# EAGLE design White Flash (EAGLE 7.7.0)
DESIGNER: A. Stummer; GROUP: R. Marjoribanks Labs; RELEASE_DATE: 2017 July; REV: A; TITLE: White Flash
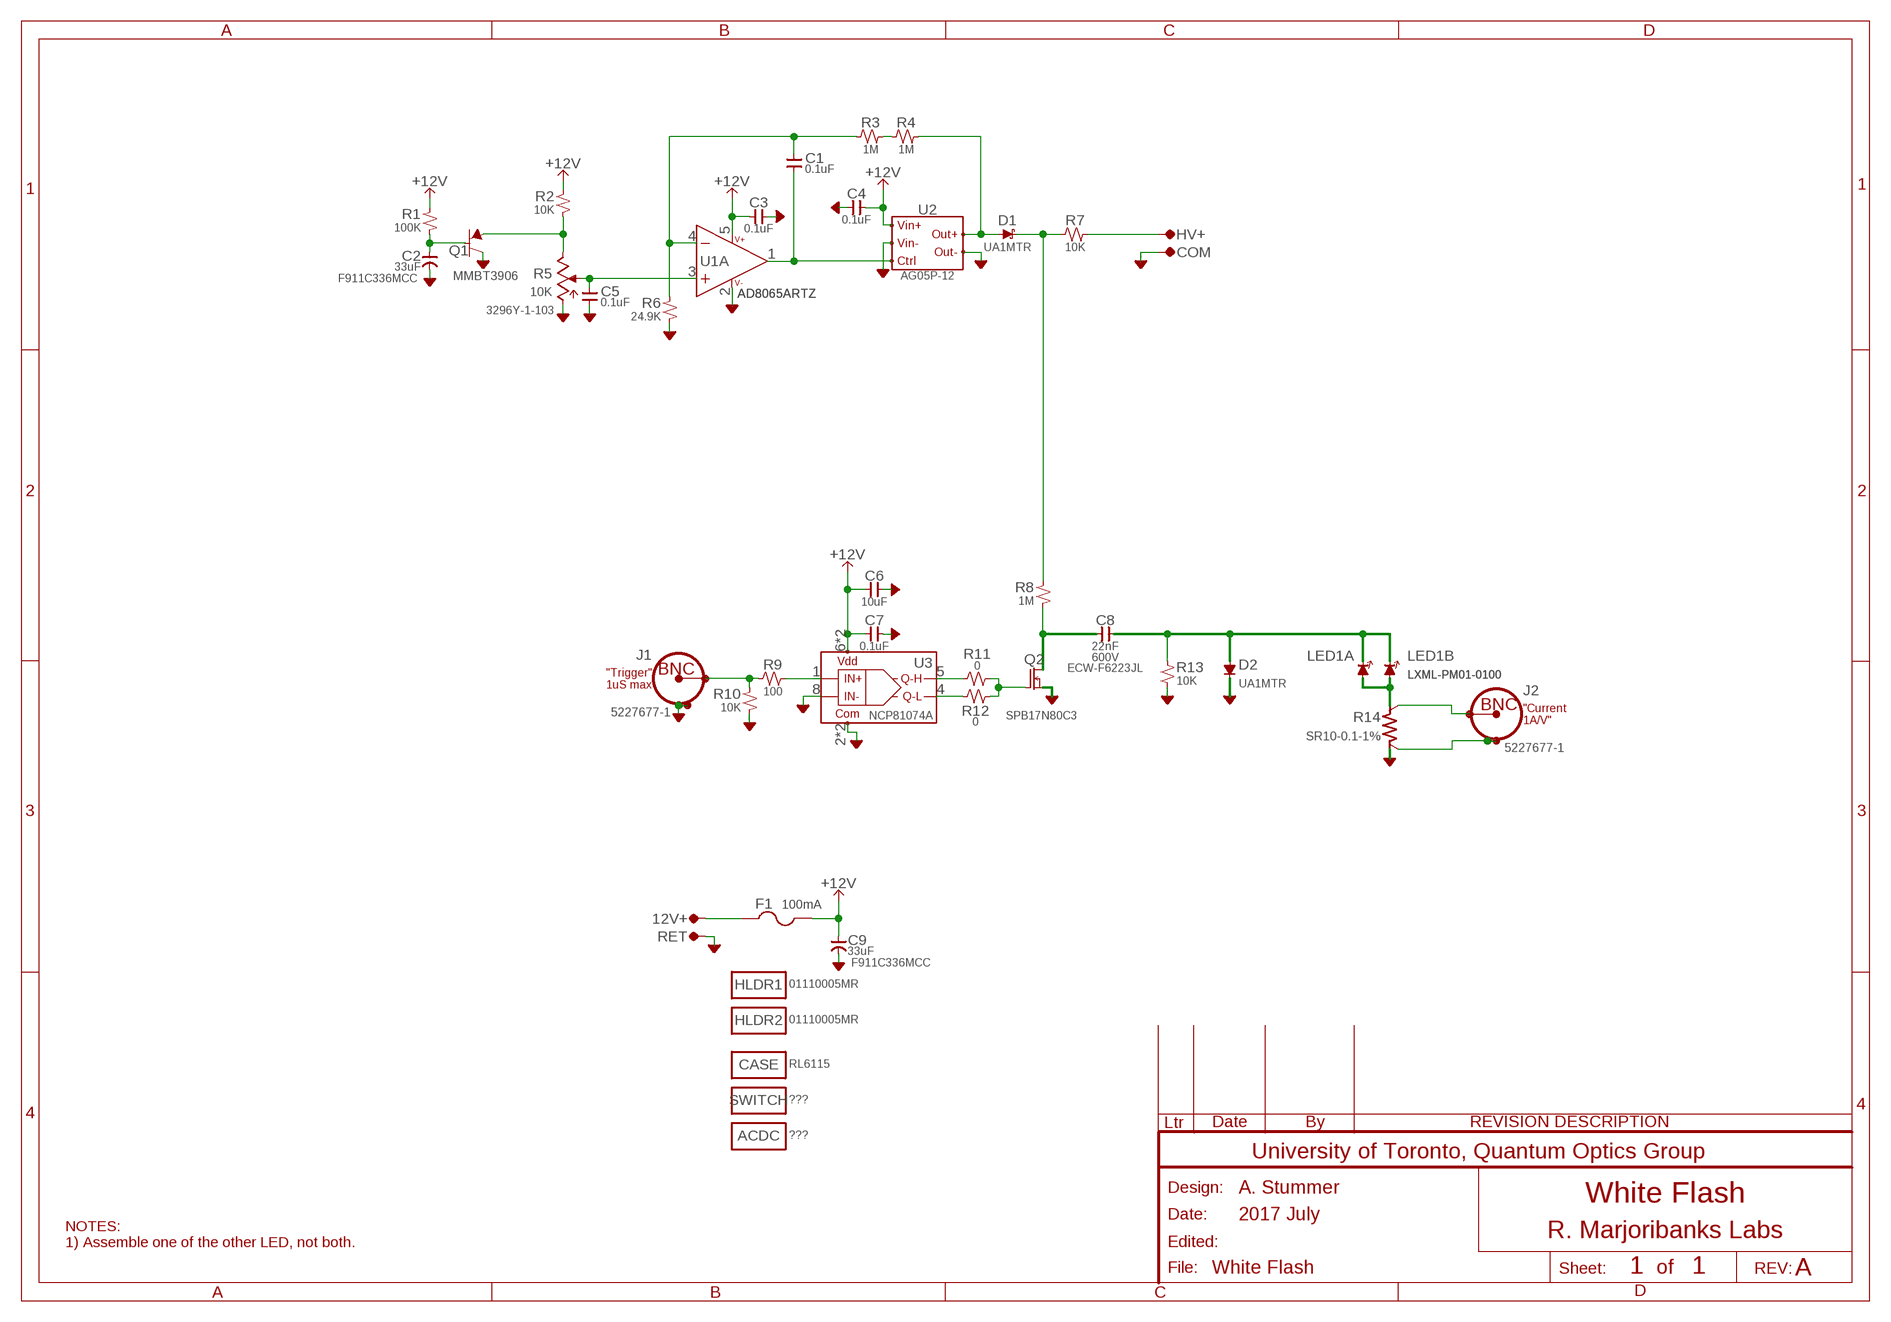
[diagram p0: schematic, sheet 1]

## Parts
12V+  TP-0.042B  [TP-0.042B]
ACDC  ???  MISC  [MISC]
C1  0.1uF  CAP-V-0805  [2012(0805)]
C2  33uF  CAP-POL--NICHICON_F91_C  [CAP:NICHICON_F91_C]
C3  0.1uF  CAP-H-0805  [2012(0805)]
C4  0.1uF  CAP-H-0805  [2012(0805)]
C5  0.1uF  CAP-V-0805  [2012(0805)]
C6  10uF  CAP-H-0805  [2012(0805)]
C7  0.1uF  CAP-H-0805  [2012(0805)]
C8  22nF  CAP-H--PASSIVE,10MM  [PASSIVE_10MM]
C9  33uF  CAP-POL--NICHICON_F91_C  [CAP:NICHICON_F91_C]
CASE  RL6115  MISC  [MISC]
COM  TP-0.042B  [TP-0.042B]
D1  UA1MTR  DIODE,SCHOTTKY-SMA  [EIA-A(SMA)]
D2  UA1MTR  DIODE,GENERIC-SMA  [EIA-A(SMA)]
F1  100mA  FUSE-5X20-4  [FUSE]
HLDR1  01110005MR  MISC  [MISC]
HLDR2  01110005MR  MISC  [MISC]
HV+  TP-0.042B  [TP-0.042B]
J1  5227677-1  CONN:BNCTYPE3HORIZ  [CONN:BNC-AMP-TYPE3HORIZ]
J2  5227677-1  CONN:BNCTYPE3HORIZ  [CONN:BNC-AMP-TYPE3HORIZ]
LED1A  LXML-PM01-0100  LED-LUMILED_REBEL  [LED_LUMILED_REBEL]
LED1B  LXML-PM01-0100  LED-LUMILED_REBEL  [LED_LUMILED_REBEL]
Q1  MMBT3906  BJT-PNP-SOT23  [SOT23]
Q2  SPB17N80C3  MOSFET-N-TO263  [TO263]
R1  100K  R-V-0805  [2012(0805)]
R2  10K  R-V-0805  [2012(0805)]
R3  1M  R-H-0805  [2012(0805)]
R4  1M  R-H-0805  [2012(0805)]
R5  10K  POT-BOURNS_3296Y  [BOURNS:3296Y]
R6  24.9K  R-V-0805  [2012(0805)]
R7  10K  R-H-0805  [2012(0805)]
R8  1M  R-V-0805  [2012(0805)]
R9  100  R-H-0805  [2012(0805)]
R10  10K  R-V-0805  [2012(0805)]
R11  0  R-H-0805  [2012(0805)]
R12  0  R-H-0805  [2012(0805)]
R13  10K  R-V-0805  [2012(0805)]
R14  SR10-0.1-1%  R-SENSE-CADDOCK_SR10  [RESISITOR,CURRENTSENSE,CADDOCK_SR10]
RET  TP-0.042B  [TP-0.042B]
SWITCH  ???  MISC  [MISC]
U1  AD8065ARTZ  OPAMP-SOT23-5  [SOT23-5]
U2  AG05P-12  DC-DC,AG-SERIES-AG(TO2KV)  [DC-DC,AG-SERIES(TO2KV)]
U3  NCP81074A  LOGIC,FET_DRIVER(NCP81074)-SOIC8  [SOIC-8]

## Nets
+12V: C3.2 C4.2 C6.1 C7.1 C9.+(POS) F1.2A F1.2B(2A) R1.2 R2.2 U1.5(B:V++) U2.IN+ U3.6(VDD) U3.7(VDD)
AGND: C2.-(NEG) C3.1 C4.1 C5.1 C6.2 C7.2 C9.-(NEG) COM.TP D2.K(C) J1.SHIELD1 J1.SHIELD2 Q1.2(E) Q2.3(S) R5.CCW R6.1 R10.1 R13.1 R14.CUR2(CURRENT2) RET.TP U1.2(B:V-) U2.HV-(OUT-) U2.IN- U3.2(COM) U3.3(COM) U3.8(IN-)
N$1: R11.1 U3.5(Q-H)
N$2: R9.2 U3.1(IN+)
N$3: J1.CONDUCTOR R9.1 R10.2
N$4: R12.1 U3.4(Q-L)
N$5: Q2.1(G) R11.2 R12.2
N$6 [HV]: D1.K(C) R7.1 R8.2
N$7 [power]: C8.1 Q2.2(D) Q2.4(D) R8.1
N$8: C1.2 R3.1 R6.2 U1.4(A:-IN)
N$9 [HV]: D1.A R4.2 U2.HV+(OUT+)
N$10: C1.1 U1.1(A:OUT) U2.CTRL
N$12: C5.2 R5.W U1.3(A:+IN)
N$13: Q1.3(C) R2.1 R5.CW
N$14: C2.+(POS) Q1.1(B) R1.1
N$15 [power]: C8.2 D2.A LED1A.K(C) LED1B.K(C) R13.2
N$16 [HV]: HV+.TP R7.2
N$17 [Pwr-LV]: LED1A.A LED1B.A R14.CUR1(CURRENT1)
N$18 [HV]: R3.2 R4.1
N$19 [Pwr-LV]: J2.CONDUCTOR R14.SEN1(SENSE1)
N$20: J2.SHIELD1 J2.SHIELD2 R14.SEN2(SENSE2)
N$22: 12V+.TP F1.1A F1.1B(1A)

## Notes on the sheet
- "Trigger"
  1uS max
- "Current
  1A/V"
- NOTES:
  1) Assemble one of the other LED, not both.

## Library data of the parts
12V+ COM HV+ RET = QuantumOptics:TP: Testpoint, single pin or single socket, either SMT pad, small hole or loop style TP such as Keystone 5002K (0.042").
ACDC CASE HLDR1 HLDR2 SWITCH = QuantumOptics:MISC: Miscellaneous Part, just a placeholder for miscellaeous parts
C1 C5 = QuantumOptics:CAP-V-: Cap, SMT and Through-hole, 0402 and up.
C2 C9 = QuantumOptics:CAP-POL-: Capacitor, Polarized, SMT 0805 and up, probably tantalum.; PN: F911C336MCC
C3 C4 C6 C7 = QuantumOptics:CAP-H-: Cap, SMT and Through-hole, 0402 and up.
C8 = QuantumOptics:CAP-H-: Cap, SMT and Through-hole, 0402 and up.; PN: ECW-F6223JL; V: 600V
D1 = QuantumOptics:DIODE,SCHOTTKY: Schottky Diode, general purpose.
D2 = QuantumOptics:DIODE,GENERIC: Diode, Generic, plain old vanilla diodes.
F1 = QuantumOptics:FUSE: Fuse
J1 J2 = QuantumOptics:CONN:BNC: BNC PCB, horizontal or vertical, e.g. Horiz: Amp (5)227677-1, nut 1-329631-2, shoulder washer 330620, vert isolated 5227222-6, http://catalog.tycoelectronics.com/TE/bin/TE.Connect?C=1&M=BYPN&TCPN=5227222-6&RQPN=5227222-6 ...
LED1A LED1B = QuantumOptics:LED: LED or laser
Q1 = QuantumOptics:BJT-PNP: PNP BJT, generic, p/n defined by VALUE field. E.g. Fairchild MMBT3906 (abs max 40V, 200mA. hFE>80@10mA.
Q2 = QuantumOptics:MOSFET-N: Mosfet, N-Channel, generic enhancement mode N-FET, such as 2N7002 in SOT-23.
R1 R2 R6 R8 R10 R13 = QuantumOptics:R-V-*: Resistor, SMT & Through-Hole, vertical symbol
R3 R4 R7 R9 R11 R12 = QuantumOptics:R-H-*: Resistor, SMT & Through-Hole, horizontal symbol
R5 = QuantumOptics:POT: Pot, regular or trimpot; PN: 3296Y-1-103
R14 = QuantumOptics:R-SENSE: Current sense resistor, 4-terminal. e.g. Ohmite series 60, http://www.ohmite.com/cgi-bin/showpage.cgi?product=60-4_series
U1 = QuantumOptics:OPAMP: Op Amp, generic, pick the right package. e.g. AD8605: SOT-23-5, RRIO, 10MHz, Ib = 1pA, Vio < 65uV, 2.7-5.5V.
U2 = QuantumOptics:DC-DC,AG-SERIES: DC-DC converter, HV #1, based on XP-Emco AG series, 100V-6KV, 1-1.5W
U3 = QuantumOptics:LOGIC,FET_DRIVER(NCP81074): FET Driver, based on NCP81074A/B, 10A 4nS

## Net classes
0 default: width 0.203 mm, drill 0.508 mm, clearance 0.203 mm
1 power: width 2.54 mm, drill 0.508 mm, clearance 2.032 mm
2 HV: width 0.203 mm, drill 0.508 mm, clearance 2.032 mm
3 Pwr-LV: width 2.54 mm, drill 0.508 mm, clearance 0.508 mm

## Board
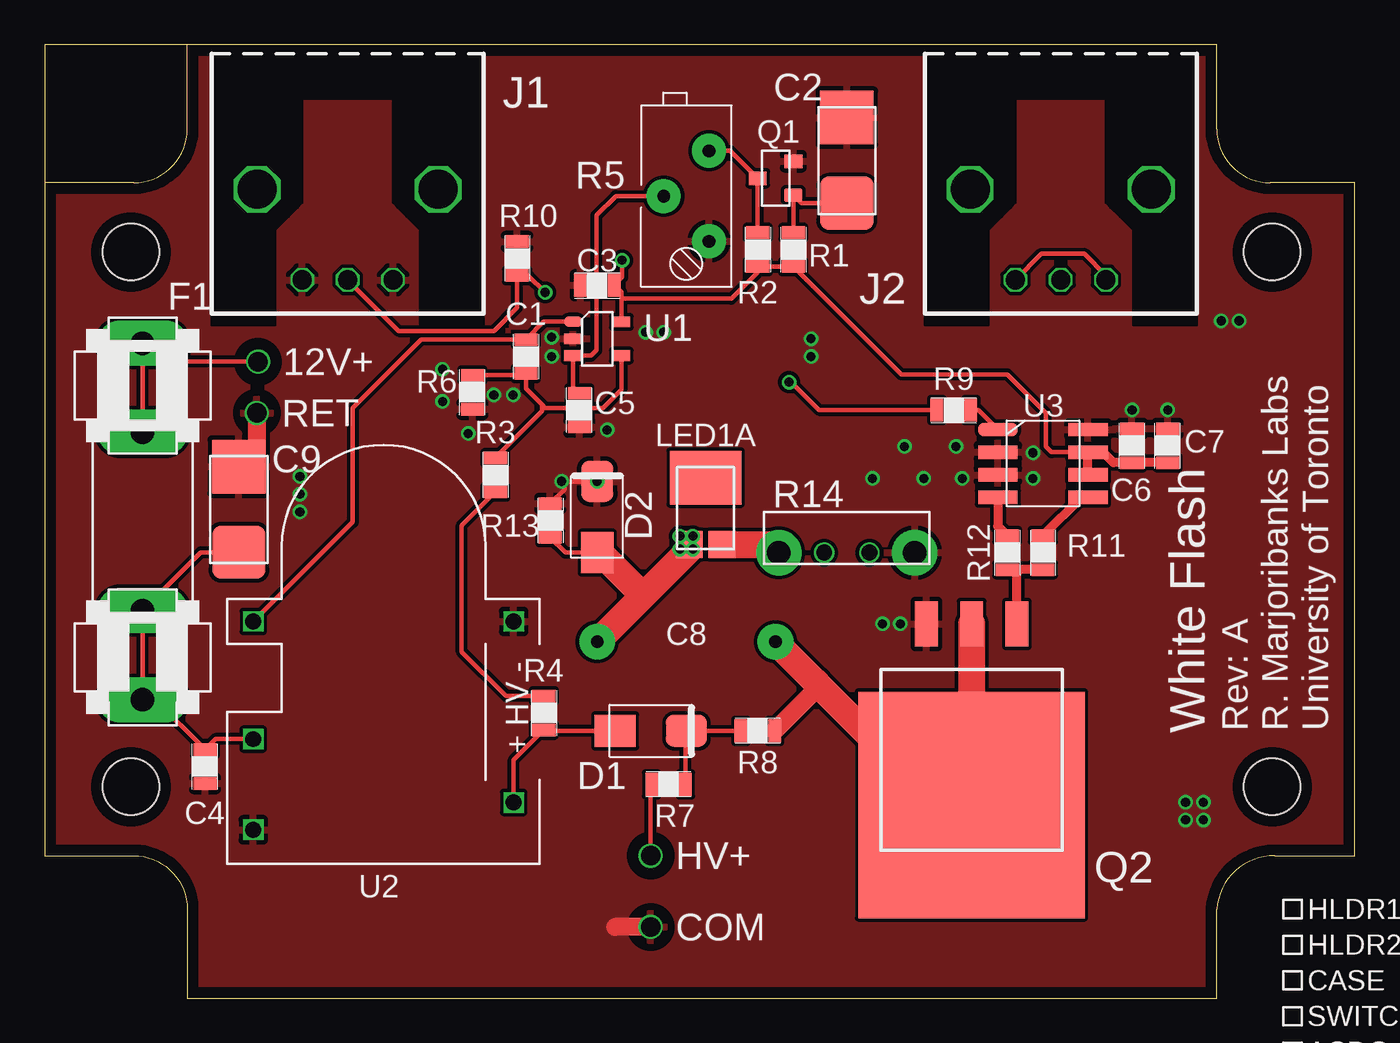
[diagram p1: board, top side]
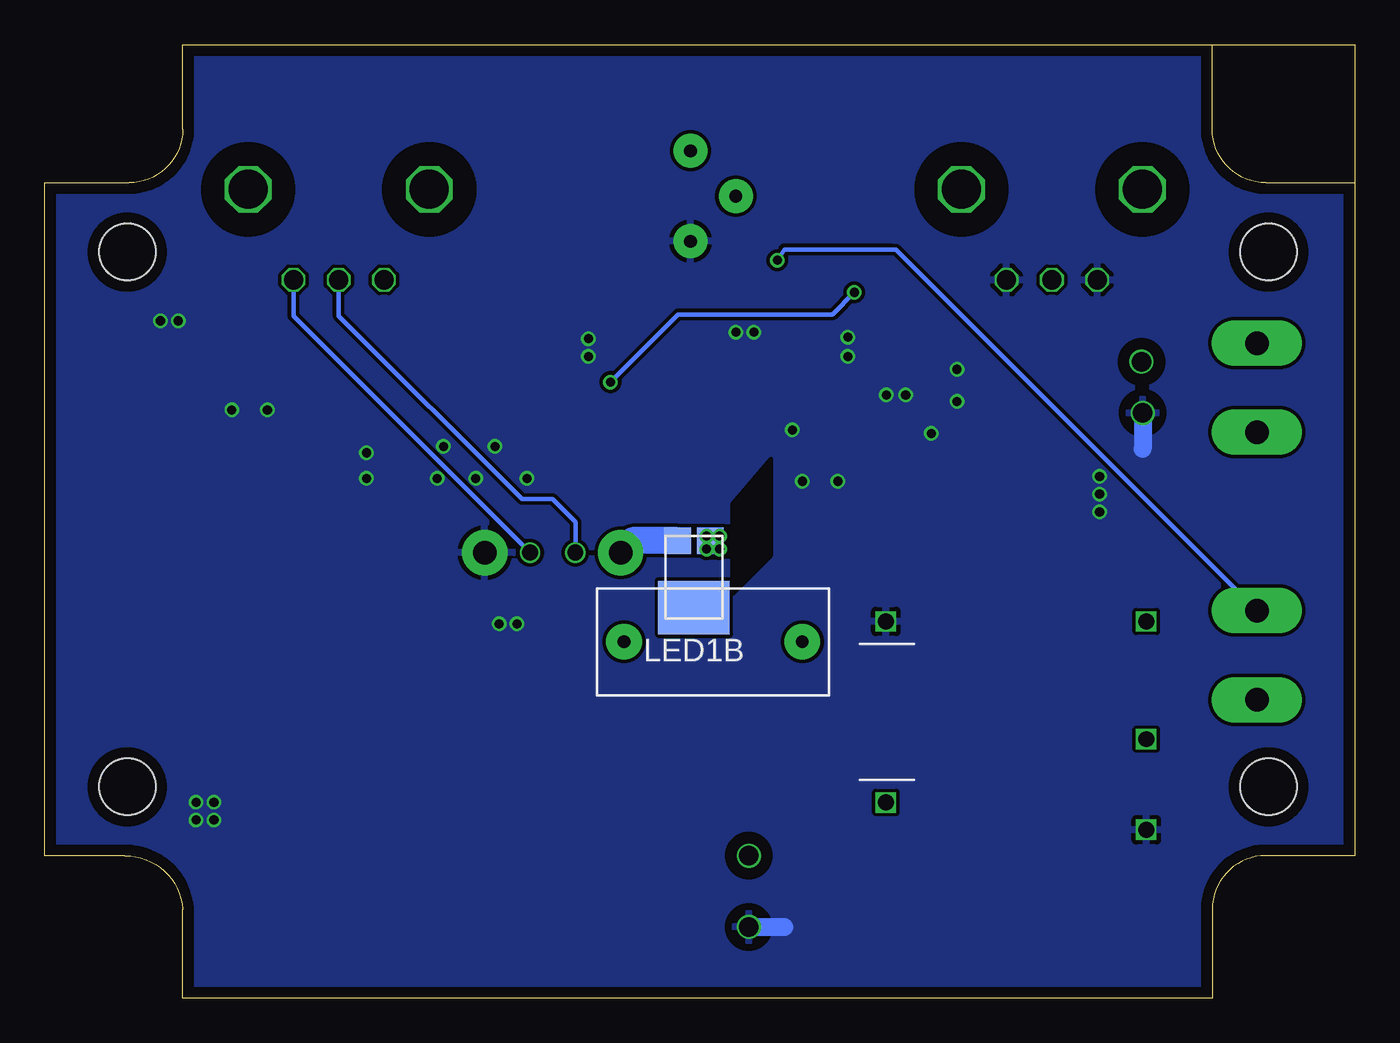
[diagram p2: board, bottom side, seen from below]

Size 73.5 x 53.5 mm. Coordinates in mm from the lower left corner, seen from the top.
Outline: 0,45.75 0,53.5 65.75,53.5 65.75,48.75 arc90 68.75,45.75 73.5,45.75 73.5,8 69,8 arc86 65.75,5 65.75,0 8,0 8,5 arc90 5,8 0,8 0,45.75
Outline: 8,53.5 8,48.75 arc-90 5,45.75 0,45.75
Copper layers (1+16): Top 0.035mm / dielectric 1.5mm / Bottom 0.035mm
Design rules "~DRC for APC, 2-layer": minimum track width 0.18mm, minimum drill 16mil, track to track 0.18mm, track to pad 0.18mm, pad to pad 0.18mm, via to via 0.18mm, smd to smd 0mil, copper to edge 25mil, drill to drill 5mil, minimum pad ring 5mil, minimum via ring 6mil, stop-mask expansion 4mil, vias tented up to drill 0mil, thermal gap 10mil
Holes 3.17 mm at 4.85,11.86 4.85,41.86 68.86,41.86 68.86,11.86
bRestrict: area 32.8,22.7 to 34.9,30.2

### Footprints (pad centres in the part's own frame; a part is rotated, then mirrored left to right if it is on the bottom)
TP-0.042B = drill 1.092: TP 0,0
2012(0805) = smd 0.7 x 1.3: 1 -0.95,0; 2 0.95,0
CAP:NICHICON_F91_C = smd 3 x 3: + -2.4,0; - 2.4,0
PASSIVE_10MM = drill 0.711 pad 2: 1 -5,0; 2 5,0
EIA-A(SMA) = smd 2.3 x 1.8: A -2,0; K 2,0
FUSE = drill 1.321 pad 2.54 long: 1A -10,0; 1B -5,0; 2A 10,0; 2B 5,0
CONN:BNC-AMP-TYPE3HORIZ = drill 1.067 octagon: CONDUCTOR 0,-12.7; SHIELD1 -2.54,-12.7; SHIELD2 2.54,-12.7 | drill 2.184 octagon: P$1 -5.08,-7.62; P$2 5.08,-7.62
LED_LUMILED_REBEL = smd 1.5 x 1.5: A 0.92,0.25; K -0.92,0.25 | smd 4 x 3: THERM 0,4
SOT23 = smd 0.75 x 1: 1 -0.95,-1; 2 0.95,-1; 3 0,1
TO263 = smd 1.27 x 2.54: 1 -2.54,0; 2 0,0; 3 2.54,0 | smd 12.7 x 12.7: 4 0,10.16
BOURNS:3296Y = drill 0.711 pad 1.905: CCW 2.54,1.27; CW -2.54,1.27; W 0,-1.27
RESISITOR,CURRENTSENSE,CADDOCK_SR10 = drill 1.321 pad 2.54: CUR1 -3.81,0; CUR2 3.81,0 | drill 0.889: SEN1 -1.27,0; SEN2 1.27,0
SOT23-5 = smd 0.6 x 1: 1 -0.95,-1.35; 2 0,-1.35; 3 0.95,-1.35; 4 0.95,1.35; 5 -0.95,1.35
DC-DC,AG-SERIES(TO2KV) = drill 0.889 square: CTRL 0,7.303; HV+ -10.16,-7.303; HV- 0,-7.303; IN+ -6.604,7.303; IN- -11.684,7.303
SOIC-8 = smd 0.75 x 2.2: 1 -1.905,-2.532; 2 -0.635,-2.532; 3 0.635,-2.532; 4 1.905,-2.532; 5 1.905,2.532; 6 0.635,2.532; 7 -0.635,2.532; 8 -1.905,2.532

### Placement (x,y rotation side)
12V+  11.97,35.71 0 top
ACDC  70,-3 0 top
C1  27,36 270 top
C2  45,47 90 top
C3  31,40 0 top
C4  9,13 90 top
C5  30,33 90 top
C6  61,31 90 top
C7  63,31 90 top
C8  36,20 0 bottom
C9  10.9,27.42 90 top
CASE  70,1 0 top
COM  34,4 0 top
D1  34,15 0 top
D2  31,27 90 top
F1  5.5,26.75 270 top
HLDR1  70,5 0 top
HLDR2  70,3 0 top
HV+  34,8 0 top
J1  17,53 0 top
J2  57,53 0 top
LED1A  37.08,25.2 0 top
LED1B  37.08,25.92 180 bottom
Q1  41,46 90 top
Q2  52,21 180 top
R1  42,42 270 top
R2  40,42 270 top
R3  25.28,29.36 270 top
R4  28,16 270 top
R5  36,45 270 top
R6  24,34 90 top
R7  35,12 180 top
R8  40,15 180 top
R9  51,33 0 top
R10  26.5,41.5 270 top
R11  56,25 270 top
R12  54,25 270 top
R13  28.36,26.8 270 top
R14  45,25 0 top
RET  11.91,32.83 0 top
SWITCH  70,-1 0 top
U1  31,37 270 top
U2  19.01,21.14 90 top
U3  56,30 270 top
U$24  [CASE,HAMMOND_RL6105_RL6115]  0,0 90 bottom

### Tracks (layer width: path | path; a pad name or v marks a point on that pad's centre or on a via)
+12V  (via drill 0.51)
  Top 0.254: U1.5 32.35,39.24 | 32.35,39.24 32.35,39.6 C3.2 32.4,40.45 v32.4,41.4 | 32.35,39.24 38.52,39.24 40,40.72 R2.2 R1.2 48.05,35 54,35 56.16,32.84 56.16,30.96 56.48,30.64 U3.7 | U2.IN+ 9.59,14.54 C4.2 6.2,16.75 F1.2A F1.2B 8.77,25.02 C9.+
  Top 0.5: U3.6 U3.7 58.57,30.6 59.4,30.6 59.95,30.05 C6.1 C7.1
  Bottom 0.25: 20.15,36.4 25.75,42 26,42
  Bottom 0.254: F1.2B 20.15,36.4 | 26,42 32,42 v32.4,41.4
AGND  (via drill 0.51)
  Top 0.254: 11.91,30.83 C9.- | R13.1 29.16,28.55 29.16,28.8 29.36,29 D2.K
  Top 1: COM.TP 32,4 | RET.TP 11.91,30.83
  Bottom 1: RET.TP 11.91,30.83 | COM.TP 32,4
  other vias: 43,36 43,37 48,21 47,21 61,33 63,33 55.44,30.6 55.44,29.16 51.48,29.16 51.12,30.96 49.32,29.16 46.44,29.16 48.24,30.96 65,10 65,11 64,11 64,10 66,38 67,38 31,29 31.56,31.88 29,29 33.72,37.36 34.72,37.36 28.44,37.08 28.44,36 22.32,35.28 22.32,33.48 25.2,33.84 26.28,33.84 23.76,31.68 14.32,29.28 14.32,28.28 14.32,27.28
  pour Bottom: 0,0 73.5,0 73.5,53.5 0,53.5
  pour Top: 0,0 73.5,0 73.5,53.5 0,53.5
N$1
  Top 0.5: U3.5 58.15,28.09 R11.1
N$2
  Top 0.254: R9.2 52.37,33 U3.1
N$3  (via drill 0.51)
  Top 0.254: 26.37,40.68 R10.2 | R10.2 27.13,40.55 v28.08,39.6 | R9.1 43.44,33 41.88,34.56 v41.76,34.56 | J1.CONDUCTOR 19.86,37.44 25.2,37.44 26.5,38.74 R10.2
  Bottom 0.254: v28.08,39.6 29.32,38.36 37.96,38.36 v41.76,34.56
N$4
  Top 0.5: U3.4 53.47,26.48 R12.1
N$5
  Top 0.5: R11.2 54.72,24.05 | 54.72,24.05 R12.2 | Q2.1 54.54,23.87 54.72,24.05
N$6
  Top 0.254: R7.1 35.95,14.95 D1.K R8.2
N$7
  Top 1: 50.16,10.84 Q2.4 | R8.1 43.28,17.33 43.28,17.72
  Top 1.5: C8.1 43.28,17.72 50.16,10.84 | Q2.2 Q2.4
N$8
  Top 0.254: U1.4 32.35,34.15 31.32,33.12 28.08,33.12 27.9,33.3 | 27.9,33.3 27,34.2 C1.2 26.9,34.95 R6.2 | R3.1 27.9,32.93 27.9,33.3
N$9
  Top 0.254: D1.A 28.05,15 R4.2 26.31,13.36 U2.HV+
N$10
  Top 0.254: U1.1 28,37.95 C1.1 21.11,36.95 17.28,33.12 17.28,26.71 U2.CTRL
N$12
  Top 0.254: C5.2 29.65,34.3 U1.3 30.65,36.05 30.96,36.36 30.96,43.92 32.04,45 R5.W
N$13
  Top 0.254: R5.CW 38.46,47.54 Q1.3 R2.1
N$14
  Top 0.254: C2.+ 42.45,44.6 Q1.1 R1.1
N$15  (via drill 0.51)
  Top 0.25: 33.12,23.04 33.58,22.58 | 36.16,25.16 LED1A.K 36.16,25.76 v35.64,25.92 v36.36,25.92 | 35.92,24.92 v35.64,25.2 v36.36,25.2
  Top 0.254: R13.2 29.21,25 D2.A
  Top 1: D2.A 31,24.8
  Top 1.5: 36.16,25.16 35.92,24.92 33.58,22.58 C8.2 | 31,24.8 31.36,24.8 33.12,23.04
  Bottom 0.25: v35.64,25.92 35.64,26.19 LED1B.K
N$16
  Top 0.254: HV+.TP 34,11.95 R7.2
N$17
  Top 1.5: LED1A.A 40.74,25.45 R14.CUR1
  Bottom 1.5: LED1B.A 40.52,25.67 R14.CUR1
N$18
  Top 0.254: R4.1 25.89,16.95 23.4,19.44 23.4,26.53 R3.2
N$19
  Bottom 0.25: 57,38.27 46.73,28 45,28 43.73,26.73 R14.SEN1
  Bottom 0.254: 57,38.27 J2.CONDUCTOR
N$20
  Top 0.254: J2.SHIELD1 55.92,41.76 58.32,41.76 59.54,40.54 J2.SHIELD2
  Bottom 0.254: R14.SEN2 59.54,38.27 J2.SHIELD2
N$22
  Top 0.254: F1.1B 5.5,35.64 | 5.5,35.64 F1.1A | 12V+.TP 5.57,35.71 5.5,35.64

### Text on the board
tNames: White Flash | Rev: A / R. Marjoribanks Labs / University of Toronto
